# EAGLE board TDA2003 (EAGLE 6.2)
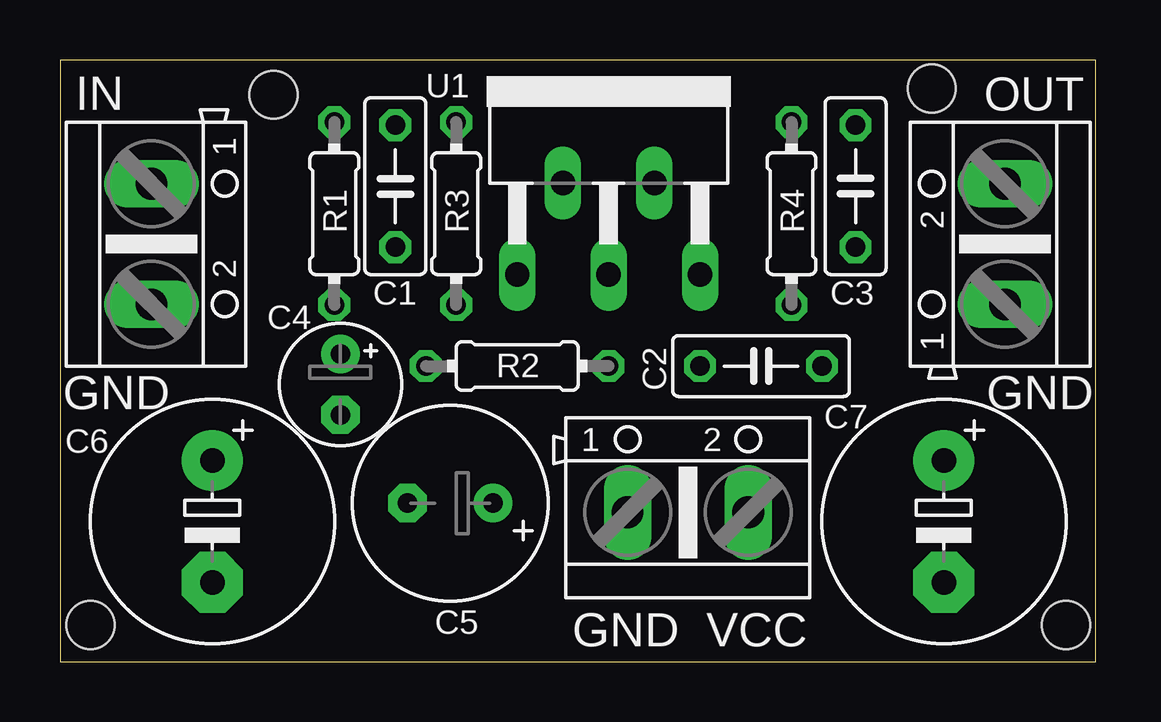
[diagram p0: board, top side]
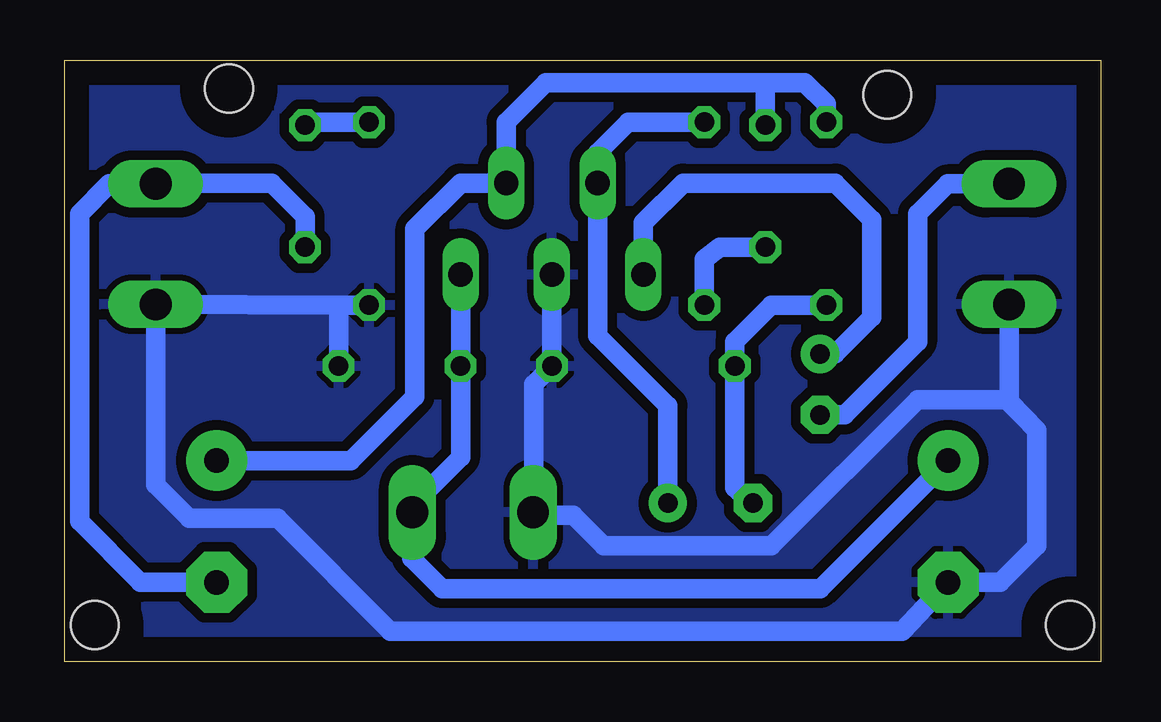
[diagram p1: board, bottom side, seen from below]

Size 43.16 x 25.07 mm. Coordinates in mm from the lower left corner, seen from the top.
Outline: 0,0 43.16,0 43.16,25.07 0,25.07 0,0
Copper layers (1*16): Top 0.035mm / dielectric 1.5mm / Bottom 0.035mm
Design rules: minimum track width 10mil, minimum drill 24mil, track to track 8mil, track to pad 8mil, pad to pad 8mil, via to via 8mil, smd to smd 8mil, copper to edge 40mil, drill to drill 8mil, minimum pad ring 10mil, minimum via ring 8mil, stop-mask expansion 4mil, vias tented up to drill 0mil, thermal gap 10mil
Holes 2 mm at 1.27,1.52 41.91,1.52 36.32,23.88 8.89,23.62

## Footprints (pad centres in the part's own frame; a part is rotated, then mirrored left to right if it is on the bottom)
C050-025X075 = drill 0.813 octagon: 1 -2.54,0; 2 2.54,0
E2,5-5 = drill 0.813 pad 1.6: + -1.27,0 | drill 0.813 pad 1.6 octagon: - 1.27,0
E3,5-8 = drill 0.813 pad 1.6: + -1.778,0 | drill 0.813 pad 1.6 octagon: - 1.778,0
E5-10,5 = drill 1.016 pad 2.54: + -2.54,0 | drill 1.016 pad 2.54 octagon: - 2.54,0
AK500/2 = drill 1.321 long: 1 -2.515,0; 2 2.515,0
0204/7 = drill 0.813 octagon: 1 -3.81,0; 2 3.81,0
CB360 = drill 1.016 long: 1 -3.81,-8.255; 2 -1.905,-4.445; 3 0,-8.255; 4 1.905,-4.445; 5 3.81,-8.255

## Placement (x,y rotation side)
C1  10nF  [C050-025X075]  13.97,19.81 270 top
C2  100nF  [C050-025X075]  29.21,12.32 0 top
C3  100nF  [C050-025X075]  33.15,19.81 90 top
C4  10uF  [E2,5-5]  11.68,11.56 270 top
C5  470uF  [E3,5-8]  16.26,6.6 180 top
C6  1000uF  [E5-10,5]  6.35,5.84 270 top
C7  1000uF  [E5-10,5]  36.83,5.84 270 top
IN  [AK500/2]  3.81,17.4 270 top
OUT  [AK500/2]  39.37,17.4 90 top
R1  470  [0204/7]  11.43,18.67 270 top
R2  4,7  [0204/7]  19.05,12.32 0 top
R3  100  [0204/7]  16.51,18.67 270 top
R4  1  [0204/7]  30.48,18.67 90 top
U1  TDA2003V  [CB360]  22.86,24.38 0 top
VCC  [AK500/2]  26.16,6.22 0 top

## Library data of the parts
C1-C7 R1-R4 = rcl
IN OUT VCC = con-ptr500; OC_FARNELL: unknown; OC_NEWARK: unknown
U1 = linear

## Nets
GND: C2.2 C6.- IN.2 OUT.1 R2.2 R4.1 U1.3 VCC.1
N$1: C4.+ U1.1
N$2: C1.2 R3.2
N$3: C5.+ R3.1 U1.2
N$4: C1.1 C7.+ R1.1 U1.4
N$5: C5.- R1.2 R2.1
N$6: C3.1 C7.- OUT.2
N$7: C3.2 R4.2
N$8: C2.1 C6.+ U1.5 VCC.2
N$9: C4.- IN.1

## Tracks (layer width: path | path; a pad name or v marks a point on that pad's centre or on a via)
GND
  Bottom 0.813: 39.35,14.88 31.75,14.86 | R4.1 31.75,14.86 | 31.75,14.86 C2.2 | U1.3 R2.2 23.62,11.56 23.62,6.83 VCC.1 23.62,5.84 23.62,6.1 21.97,6.1 20.7,4.83 13.72,4.83 7.62,10.92 3.94,10.92 2.67,9.65 | OUT.1 39.37,7.37 37.97,5.97 34.29,5.97 29.59,1.27 8.26,1.27 C6.- 4.19,3.3 2.67,4.83 2.67,9.65 | 2.67,9.65 3.81,10.82 IN.2
  pour Bottom (isolate 0.406): 0,25.65 43.94,25.65 43.94,-0.38 0,-0.38
N$1
  Bottom 0.813: U1.1 19.05,18.29 17.4,19.94 11.05,19.94 9.52,18.42 9.52,14.35 11.05,12.83 C4.+
N$2
  Bottom 0.813: C1.2 15.88,17.27 16.51,16.76 R3.2
N$3
  Bottom 0.813: R3.1 19.69,22.48 20.96,21.21 U1.2 20.96,13.59 18.03,10.67 C5.+
N$4
  Bottom 0.813: 13.97,24.13 12.32,24.13 11.43,23.24 R1.1 | 13.97,24.13 23.11,24.13 24.76,22.48 24.76,20.57 | 24.76,20.57 U1.4 | C7.+ 31.24,8.38 28.57,11.05 28.57,18.03 26.67,19.94 25.4,19.94 24.76,20.57 | C1.1 13.97,24.13
N$5
  Bottom 0.813: R1.2 13.72,14.86 15.24,13.33 R2.1 15.24,7.24 14.48,6.48 C5.-
N$6
  Bottom 0.813: C7.- 40.01,3.3 42.54,5.84 42.54,18.67 41.3,19.91 OUT.2 40.11,19.94 34.54,19.94 33.15,18.54 C3.1
N$7
  Bottom 0.813: R4.2 32.89,22.48 C3.2
N$8
  Bottom 0.813: U1.5 C2.1 26.67,8.51 28.68,6.5 VCC.2 28.7,4.55 28.7,4.32 27.43,3.05 11.68,3.05 C6.+
N$9
  Bottom 0.813: IN.1 6.38,19.91 7.62,18.67 7.62,13.33 10.67,10.29 C4.-

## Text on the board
tNames: GND | GND | GND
